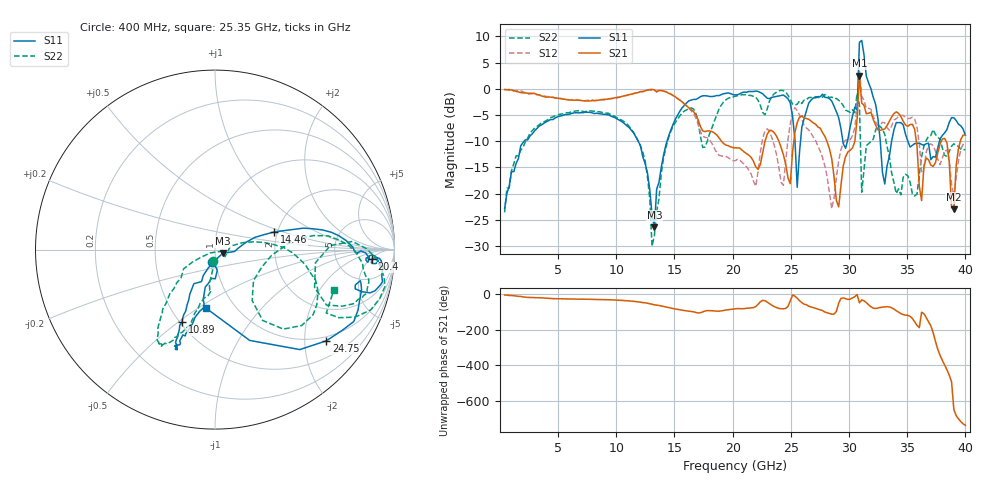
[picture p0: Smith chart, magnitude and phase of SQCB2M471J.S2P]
! Network Analyzer HP8722ES.07.66: Jul 25, 2000 Serial No. US39175408
! 27 Oct 2004  14:35:53
! Frequency  S11  S21  S12  S22
# HZ  S  DB R  50
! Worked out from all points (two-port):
!   201 points, 400 MHz to 40 GHz, reference 50 ohm
!   highest |S21| = 2.50 dB at 30.89 GHz (marker M1); lowest = -23.0 dB at 39.01 GHz (marker M2)
!   |S21| within 3 dB of the highest: start of sweep to 1.387 GHz; 12.32 GHz to 13.45 GHz (1.132 GHz wide, 8.78 % of centre)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
!   lowest |S11| = -26.5 dB at 13.27 GHz (marker M3), VSWR 1.10, Z = 54.4 - j2.27 ohm
!   |S11| at or under -10 dB: start of sweep to 2.085 GHz; 11.88 GHz to 14.36 GHz (2.482 GHz wide, 18.9 % of centre); 35.05 GHz to 37.77 GHz (2.721 GHz wide, 7.47 % of centre)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
!   |S22| runs from -30.0 to -0.3 dB; largest |S21 - S12| = 0.48
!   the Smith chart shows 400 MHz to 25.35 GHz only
!   S11 on the Smith chart (normalised r, x): 400 MHz: 0.96, -0.13; 10.89 GHz: 0.51, -0.52; 14.46 GHz: 1.92, +0.43; 20.4 GHz: 13, -6; 24.75 GHz: 0.89, -2.52; 25.35 GHz: 0.74, -0.54
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4e8  -22.87 -104.4  -0.16 -3.3  -0.11 -2.8  -23.58 -102.1
7.132e9  -4.59 -111.8  -2.30 -26.3  -2.35 -27.9  -4.34 -119.2
1.0894e10  -7.04 -114.4  -1.26 -35.3  -1.28 -36.9  -6.69 -129.6
1.327e10  -26.46 -26.0  -0.22 -58.3  -0.32 -61.1  -28.03 -13.4
1.3666e10  -17.83 3.1  -0.33 -62.0  -0.32 -64.6  -21.03 12.6
1.4458e10  -9.27 16.6  -0.81 -73.4  -0.73 -77.4  -9.60 4.7
2.02e10  -1.17 -4.8  -11.28 -81.0  -13.72 -75.8  -1.45 -9.2
2.0398e10  -1.15 -3.5  -11.29 -79.6  -13.49 -74.7  -1.35 -10.3
2.4754e10  -1.92 -39.3  -17.01 -67.3  -9.64 1.9  -1.24 -25.7
2.5348e10  -9.62 -98.6  -8.37 -9.2  -3.62 -43.1  -3.11 -18.8
2.6932e10  -1.74 22.2  -6.54 -73.7  -9.23 -88.6  -1.75 -23.6
2.8912e10  -4.39 -62.9  -21.30 -95.5  -16.95 -6.5  -1.86 -57.4
2.9902e10  -9.64 140.1  -12.07 -27.9  -9.75 -24.7  -4.29 -90.6
3.0694e10  -4.06 45.7  -5.83 -0.4  -3.27 -4.4  -0.86 -136.2
3.0892e10  8.85 47.6  2.50 -47.2  3.67 -64.9  -3.00 132.3
3.109e10  9.21 -6.8  -2.71 -30.4  -1.42 -36.1  -19.73 -98.9
3.1288e10  6.44 -37.7  -3.19 -36.2  -2.21 -40.2  -15.45 -32.2
3.2278e10  -2.91 -117.6  -6.89 -78.9  -6.30 -80.8  -7.98 -11.4
3.3466e10  -12.87 -10.9  -6.20 -70.5  -7.90 -79.2  -12.99 -143.5
3.6832e10  -10.40 -174.9  -13.54 -154.6  -10.76 -129.7  -9.09 -165.7
3.901e10  -5.54 33.4  -22.97 69.3  -20.51 123.1  -10.51 -22.5
4e10  -8.87 -21.2  -8.81 -20.4  -11.17 -13.6  -11.57 -129.4
